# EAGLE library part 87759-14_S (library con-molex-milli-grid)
HEADER
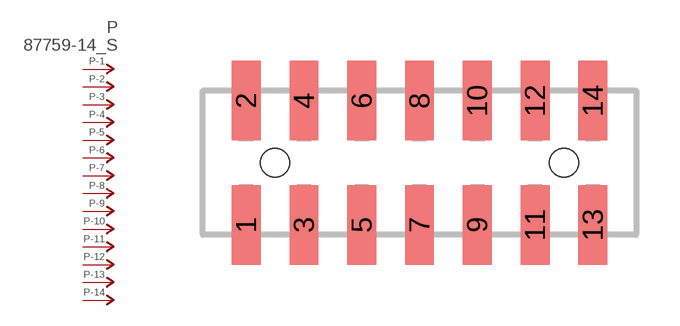
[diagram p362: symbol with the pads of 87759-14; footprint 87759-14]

Designator prefix P; gates -1=P-NV -2=P-N -3=P-N -4=P-N -5=P-N -6=P-N -7=P-N -8=P-N -9=P-N -10=P-N -11=P-N -12=P-N -13=P-N -14=P-N

## 87759-14_S  [87759-14]
1  -1:P  pas
2  -2:P  pas
3  -3:P  pas
4  -4:P  pas
5  -5:P  pas
6  -6:P  pas
7  -7:P  pas
8  -8:P  pas
9  -9:P  pas
10  -10:P  pas
11  -11:P  pas
12  -12:P  pas
13  -13:P  pas
14  -14:P  pas

## Footprint 87759-14 (pad centres in mm)
HEADER SMD Dual Row, Vertical
smd 1 x 2.75: 1 -6,-2.15; 2 -6,2.15; 3 -4,-2.15; 4 -4,2.15; 5 -2,-2.15; 6 -2,2.15; 7 0,-2.15; 8 0,2.15; 9 2,-2.15; 10 2,2.15; 11 4,-2.15; 12 4,2.15; 13 6,-2.15; 14 6,2.15
hole 1 at -5,0
hole 1 at 5,0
